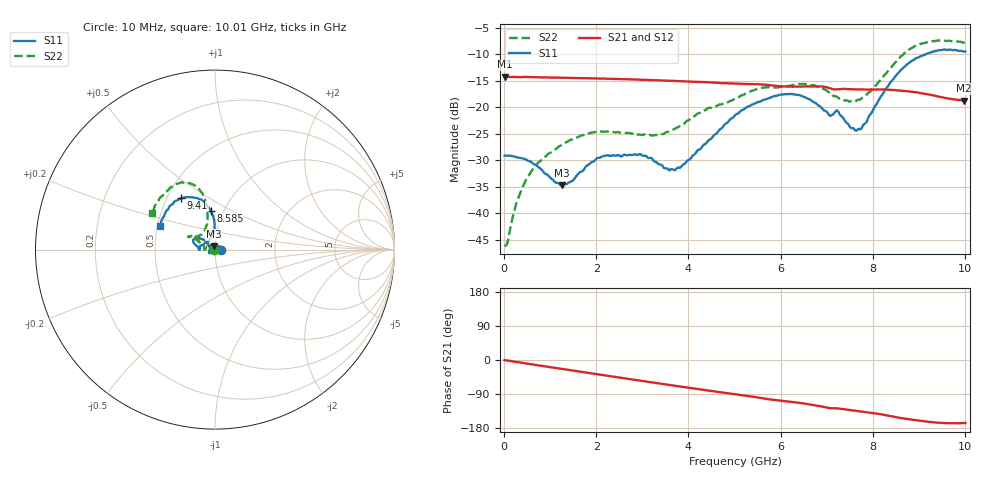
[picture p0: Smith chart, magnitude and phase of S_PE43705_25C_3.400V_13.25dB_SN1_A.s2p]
! Device ID: PE43705
! Serial: 1
! Insertion: A
! Impedance: 50 ohm
! Temp: 25C
! VDD: 3.400V
! Attenuation Step: 13.25dB
#  Hz  S  RI  R  50
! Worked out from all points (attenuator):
!   401 points, 10 MHz to 10.01 GHz, reference 50 ohm
!   highest |S21| = -14.26 dB at 10 MHz (marker M1); lowest = -18.7 dB at 9.985 GHz (marker M2)
!   lowest |S11| = -34.7 dB at 1.26 GHz (marker M3), VSWR 1.04, Z = 49.3 + j1.71 ohm
!   |S11| at or under -10 dB: start of sweep to 9.156 GHz
!   |S22| runs from -46.2 to -7.4 dB; largest |S21 - S12| = 0.0018
!   S11 on the Smith chart (normalised r, x): 10 MHz: 1.07, +0.00; 8.585 GHz: 0.87, +0.39; 9.41 GHz: 0.59, +0.38; 10.01 GHz: 0.51, +0.15
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1e7  0.0349 0.000206  0.1936 -0.000884  0.1937 -0.000843  -0.00486 0.000437
8.5e7  0.0347 0.00253  0.193 -0.00581  0.193 -0.00573  -0.00432 0.00354
2.85e8  0.032 0.00975  0.1915 -0.0184  0.1915 -0.0183  -0.00583 0.0118
5.1e8  0.0263 0.0171  0.1892 -0.0328  0.1893 -0.0326  -0.0103 0.0194
1.26e9  -0.00625 0.0173  0.1735 -0.076  0.1736 -0.0758  -0.0378 0.0228
1.685e9  -0.024 0.006  0.1603 -0.098  0.1603 -0.0979  -0.0521 0.0149
2.21e9  -0.0331 -0.0112  0.1401 -0.1218  0.1401 -0.1218  -0.0588 0.00324
2.96e9  -0.03 -0.0201  0.1048 -0.1483  0.1051 -0.1482  -0.0548 0.00307
3.36e9  -0.025 -0.0145  0.0844 -0.1578  0.0846 -0.1576  -0.0544 0.00666
3.86e9  -0.0275 0.00577  0.058 -0.1657  0.0581 -0.1656  -0.0657 0.0203
5.01e9  -0.063 0.0555  -0.0015 -0.1669  -0.00127 -0.167  -0.1063 0.0574
5.985e9  -0.1165 0.0599  -0.0464 -0.1507  -0.0455 -0.1507  -0.1357 0.0742
6.685e9  -0.1106 0.0274  -0.0742 -0.1382  -0.0743 -0.1379  -0.1445 0.0711
7.06e9  -0.083 0.00654  -0.0906 -0.1208  -0.0904 -0.1214  -0.1156 0.0742
7.235e9  -0.092 0.0121  -0.0903 -0.1167  -0.0901 -0.1168  -0.1004 0.0732
7.685e9  -0.0357 0.0511  -0.1036 -0.1041  -0.1034 -0.1043  -0.0637 0.0989
8.36e9  -0.00454 0.1657  -0.123 -0.0786  -0.1225 -0.0791  -0.0445 0.2239
8.585e9  -0.0243 0.2158  -0.1267 -0.0662  -0.1261 -0.0669  -0.0603 0.2865
8.935e9  -0.0753 0.2788  -0.1289 -0.05  -0.1286 -0.0488  -0.1189 0.3617
9.41e9  -0.1889 0.2859  -0.1226 -0.0319  -0.1221 -0.0316  -0.2189 0.3646
9.985e9  -0.3019 0.1407  -0.1123 -0.0272  -0.1124 -0.0275  -0.3455 0.2139
1.001e10  -0.3083 0.1323  -0.1128 -0.0277  -0.1131 -0.0284  -0.353 0.2031
